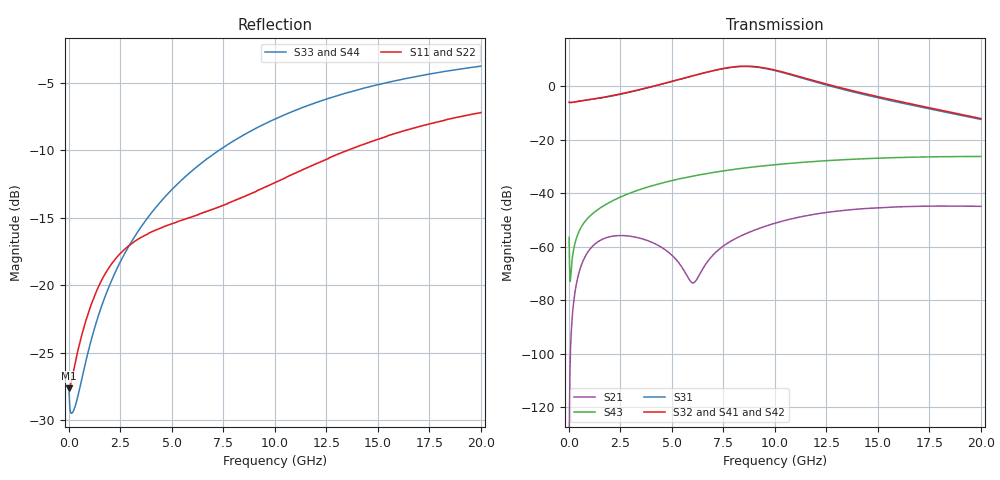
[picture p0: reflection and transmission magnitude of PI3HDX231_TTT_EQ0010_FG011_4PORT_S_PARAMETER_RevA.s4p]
! NPort=4 DATA=2000 NOISE=0 GROUPDELAY=0 COMPLEX_DATAFORMAT=POLAR
! NumOfBlock=1 NumOfParam=0
! .MODEL Smodel S TSTONEFILE=PI3HDX231_TTT_EQ0010_FG011_4PORT_S_PARAMETER_RevA.s4p TYPE=S
!  -- The above .MODEL line can be used for the S element in the netlist.
! The s parameter is extracted from the linear redriver, it is not bi-directional; only s(4,1)s(4,2) and s(3,1)s(3,2)
! should be the insertion loss
!Port definition:
!Port1 = input+
!Port2 = input-
!Port3 = output+
!Port4 = output-
# Hz S MA R  50
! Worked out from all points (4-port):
!   2000 points, 10 MHz to 20 GHz, reference 50 ohm
!   strongest paths, dB at 10 MHz, 5.01 GHz, 10.01 GHz, 15.01 GHz, 20 GHz:
!     S32: -5.9, 1.9, 6.1, -3.8, -12.0
!     S41: -5.9, 2.0, 6.1, -3.9, -12.1
!     S42: -5.9, 2.0, 6.1, -4.0, -11.9
!     S31: -5.9, 1.9, 5.9, -4.3, -12.3
!     S43: -56.5, -35.2, -29.3, -26.9, -26.2
!     S21: -134.8, -63.3, -51.2, -45.4, -44.9
!   lowest |S11| = -27.6 dB at 10 MHz (marker M1), VSWR 1.09, Z = 46 - j0.0776 ohm
!   |S11| at or under -10 dB: start of sweep to 13.55 GHz
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1e7  0.04152 -178.8  1.825e-07 -13.9  0 0.0  0 0.0
     1.825e-07 -14.0  0.04152 -178.8  0 0.0  0 0.0
     0.5041 -0.6  0.5041 179.4  0.04012 -3.2  0.0015 -70.3
     0.5041 179.4  0.5041 -0.6  0.0015 -70.3  0.04012 -3.2
1.98e9  0.1173 -139.4  0.001535 46.0  1.652e-12 -64.3  1.502e-12 -55.3
        0.001535 46.0  0.1173 -139.5  1.468e-12 -56.7  1.69e-12 -62.9
        0.6513 -7.2  0.6601 173.1  0.1003 -89.4  0.006783 73.8
        0.6615 173.2  0.6516 -6.4  0.006782 73.8  0.1003 -89.4
5.65e9  0.1758 -138.9  0.0003218 -2.5  1.13e-09 172.8  4.889e-10 -156.0
        0.0003263 -2.1  0.1757 -139.1  4.556e-10 -154.7  1.198e-09 172.7
        1.45 -60.3  1.454 119.0  0.2519 -104.4  0.0197 58.0
        1.459 118.8  1.476 -59.1  0.01965 57.9  0.252 -104.4
7.62e9  0.1995 -134.4  0.001115 101.0  7.66e-09 109.4  3.104e-09 -178.5
        0.00111 100.2  0.199 -134.6  2.993e-09 -175.2  8.136e-09 108.1
        2.201 -115.7  2.218 63.8  0.328 -109.7  0.02677 46.0
        2.221 63.5  2.248 -114.5  0.02667 46.0  0.3282 -109.7
9.12e9  0.223 -131.1  0.00213 90.4  2.025e-08 58.1  1.297e-08 139.4
        0.002116 89.9  0.2221 -131.3  1.27e-08 142.1  2.138e-08 55.8
        2.297 -171.7  2.336 7.8  0.3819 -113.5  0.03172 36.2
        2.334 7.5  2.348 -170.4  0.03161 36.3  0.3821 -113.5
1.127e10  0.2654 -128.4  0.003664 70.0  4.851e-08 2.1  4.295e-08 65.0
          0.003637 69.6  0.2638 -128.5  4.23e-08 67.5  5.02e-08 -1.0
          1.452 121.1  1.501 -60.0  0.4521 -118.6  0.03789 22.2
          1.495 -60.3  1.487 122.6  0.03778 22.4  0.4522 -118.7
2e10  0.4354 -135.6  0.005737 -4.8  3.74e-07 -159.7  2.77e-07 -130.4
      0.005688 -4.9  0.4337 -135.4  2.778e-07 -128.9  3.693e-07 -162.5
      0.2415 -28.1  0.2506 145.0  0.6464 -135.0  0.04881 -32.2
      0.2483 145.3  0.2538 -26.5  0.04893 -32.0  0.6461 -135.0
